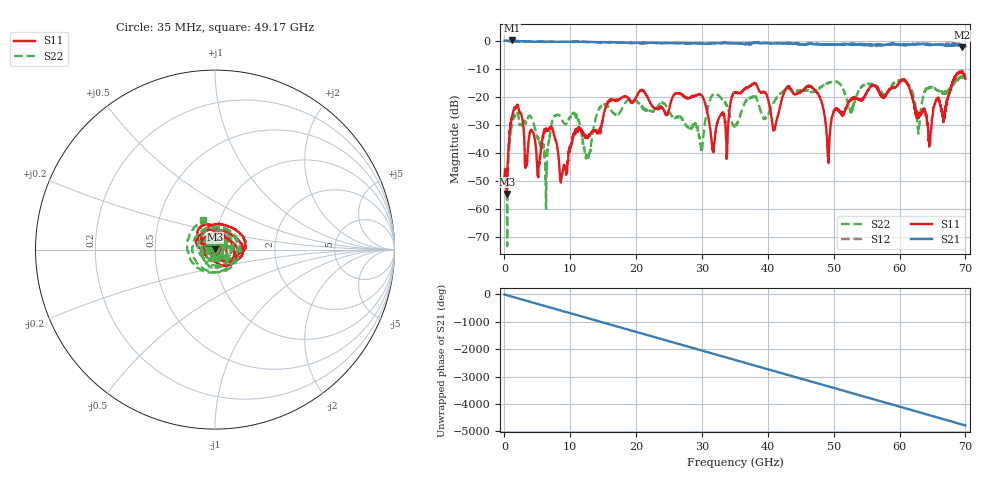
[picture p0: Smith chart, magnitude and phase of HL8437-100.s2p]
! 7/12/2021 10:41:18 AM
! H:\PROTOTYPE_DATA\DCBS_7-8-21\100NF_16V_CERAMIC_3_5880.S2P
! CHANNEL.1
! TR.MEASUREMENT
! CORRECTED.DATA
# GHZ S RI R 50.0
! FREQ.GHZ  S11RE  S11IM  S21RE  S21IM  S12RE  S12IM  S22RE  S22IM
!; PortSelection: Port_12
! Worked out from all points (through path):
!   2000 points, 35 MHz to 70 GHz, reference 50 ohm
!   highest |S21| = 0.07 dB at 1.155 GHz (marker M1); lowest = -2.3 dB at 69.55 GHz (marker M2)
!   group delay of S21, straight-line fit = 190 ps
!   lowest |S11| = -54.7 dB at 385 MHz (marker M3), VSWR 1.00, Z = 50.1 + j0.176 ohm
!   |S11| at or under -10 dB: start of sweep to end of sweep
!   |S22| runs from -73.4 to -11.9 dB; largest |S21 - S12| = 0.087
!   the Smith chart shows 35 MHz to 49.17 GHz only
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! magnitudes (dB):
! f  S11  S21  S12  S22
! 35 MHz  -48.2  0.0  0.0  -51.0
! 385 MHz  -54.7  -0.1  -0.1  -57.8
! 1.155 GHz  -27.4  0.1  0.0  -30.3
! 5.145 GHz  -48.8  -0.3  -0.4  -35.3
! 6.3 GHz  -31.4  -0.4  -0.4  -58.3
! 8.68 GHz  -48.5  -0.4  -0.4  -28.0
! 11.72 GHz  -31.8  -0.4  -0.4  -33.7
! 23.38 GHz  -24.5  -0.8  -0.9  -23.6
! 29.89 GHz  -19.3  -1.0  -0.9  -39.9
! 31.71 GHz  -39.7  -0.8  -1.0  -19.2
! 35.03 GHz  -18.4  -0.9  -0.9  -30.4
! 38.12 GHz  -15.3  -0.6  -0.7  -19.9
! 40.98 GHz  -31.6  -1.0  -1.0  -21.7
! 46.69 GHz  -16.7  -1.1  -1.1  -18.3
! 49.17 GHz  -42.1  -1.2  -1.4  -15.1
! 50.3 GHz  -24.6  -1.3  -1.4  -14.6
! 58.34 GHz  -18.1  -1.2  -1.5  -18.2
! 61.22 GHz  -15.4  -1.2  -1.4  -15.2
! 62.86 GHz  -26.3  -1.3  -1.1  -33.2
! 64.54 GHz  -35.4  -1.6  -1.3  -16.8
! 69.55 GHz  -10.9  -2.3  -1.9  -12.8
! 70 GHz  -13.7  -1.9  -1.9  -12.5
